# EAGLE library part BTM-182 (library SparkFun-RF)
Rayson BTM-182 Bluetooth Module The BTM-182 is an easy to use Bluetooth SPP (Serial Port Protocol) module, designed for transparent wireless serial connection setup. This is a fully qualified Bluetooth V2.0+EDR (Enhanced Data Rate) 3Mbps modulation with complete 2.4GHz radio transceiver. It uses CSR Bluecore 04 external single chip Bluetooth system with CMOS technology and with AFH (Adaptive Frequency Hopping). SparkFun Products: Bluetooth DIP Module - Rayson BTM-182 (WRL-9977)
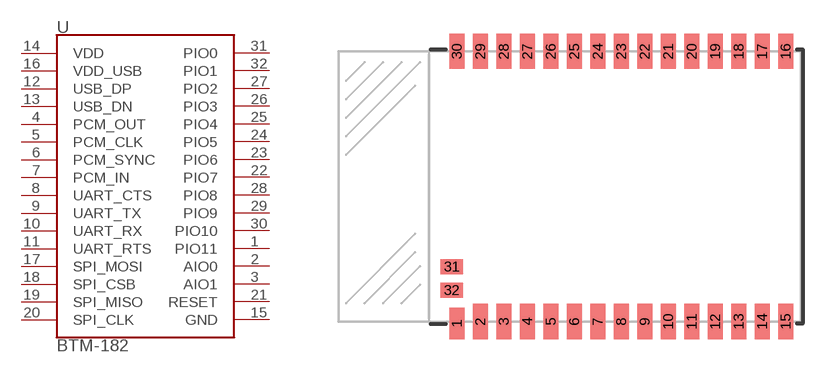
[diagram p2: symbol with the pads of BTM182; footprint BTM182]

Designator prefix U

## BTM-182_ (PROD_ID: IC-09842; SF_ID: WRL-09913)  [BTM182]
1  PIO11
2  AIO0
3  AIO1
4  PCM_OUT
5  PCM_CLK
6  PCM_SYNC
7  PCM_IN
8  UART_CTS
9  UART_TX
10  UART_RX
11  UART_RTS
12  USB_DP
13  USB_DN
14  VDD
15  GND
16  VDD_USB
17  SPI_MOSI
18  SPI_CSB
19  SPI_MISO
20  SPI_CLK
21  RESET
22  PIO7
23  PIO6
24  PIO5
25  PIO4
26  PIO3
27  PIO2
28  PIO8
29  PIO9
30  PIO10
31  PIO0
32  PIO1

## Footprint BTM182 (pad centres in mm)
Rayson BTM-182 Bluetooth Module BTM-182 Class2 Bluetooth Module from Rayson Datasheet
smd 0.8 x 1.7: 1 -6.1,-7.4
smd 0.8 x 1.9: 2 -4.83,-7.3; 3 -3.56,-7.3; 4 -2.29,-7.3; 5 -1.02,-7.3; 6 0.25,-7.3; 7 1.52,-7.3; 8 2.79,-7.3; 9 4.06,-7.3; 10 5.33,-7.3; 11 6.6,-7.3; 12 7.87,-7.3; 13 9.14,-7.3; 14 10.41,-7.3; 15 11.68,-7.3; 16 11.68,7.3; 17 10.41,7.3; 18 9.14,7.3; 19 7.87,7.3; 20 6.6,7.3; 21 5.33,7.3; 22 4.06,7.3; 23 2.79,7.3; 24 1.52,7.3; 25 0.25,7.3; 26 -1.02,7.3; 27 -2.29,7.3; 28 -3.56,7.3; 29 -4.83,7.3; 30 -6.1,7.3
smd 1.2 x 0.8: 31 -6.38,-4.34; 32 -6.38,-5.61

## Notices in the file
Licensing: Creative Commons ShareAlike 4.0 International - https://creativecommons.org/licenses/by-sa/4.0
